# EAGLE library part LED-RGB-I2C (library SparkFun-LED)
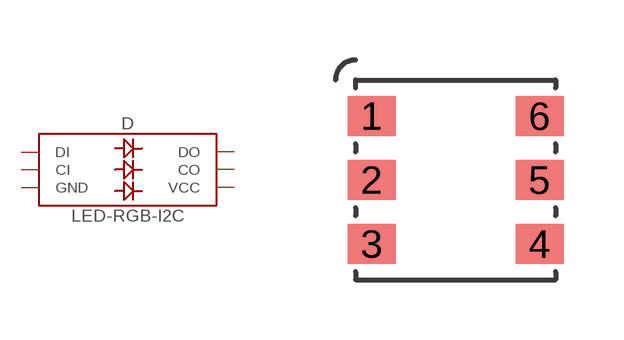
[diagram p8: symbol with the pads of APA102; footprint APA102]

Designator prefix D

## LED-RGB-I2C  [APA102]
1  DI
2  CI
3  GND
4  VCC
5  CO
6  DO

## Footprint APA102 (pad centres in mm)
smd 1.2 x 1: 1 -2.1,1.6; 2 -2.1,0; 3 -2.1,-1.6; 4 2.1,-1.6; 5 2.1,0; 6 2.1,1.6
